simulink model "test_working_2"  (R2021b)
settings: Solver=FixedStepAuto  StartTime=0.0  StopTime=Inf  FixedStep=0.01  RelTol=1e-3  EnableMultiTasking=on
undefined symbols (not defined in the file): imu, localhost, name, type, value, vel
libraries: genomix x3

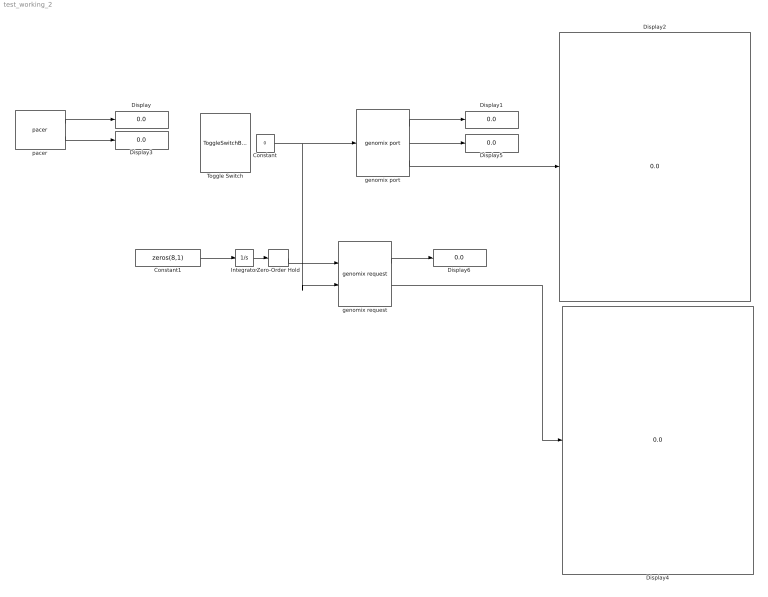
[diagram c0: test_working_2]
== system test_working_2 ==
  Constant : Constant  Value=0  OutDataTypeStr=boolean  SampleTime=-1
  Constant1 : Constant  Value=zeros(8,1)  OutDataTypeStr=double
  Display{,1..6} (7 alike) : Display
  Integrator : Integrator
  Toggle Switch : ToggleSwitchBlock
  Zero-Order Hold : ZeroOrderHold  SampleTime=-1
  genomix port : genomix/genomix port  host=localhost:20001  component=rotorcraft  instance=rotorcraft_mk3  port=imu  sigtype=value  timetype=triggered (level)  period=0.1  siglist="[{\"name\":\"imu.acc\",\"type\":\"value\",\"size\":3}]"
  genomix request : genomix/genomix request  host=localhost:20001  component=nhfc  instance=nhfc_mk3  port=set_state  sigtype=value  timetype=triggered (level)  period=Tsim  siglist="[{\"name\":\"vel\",\"type\":\"value\",\"size\":3}]"
  pacer : genomix/pacer  Priority=0  catchup=off
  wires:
  genomix port/1 -> Display1/1
  genomix port/3 -> Display2/1
  Constant/1 -> genomix request/2, genomix port/1
  pacer/1 -> Display/1
  pacer/2 -> Display3/1
  genomix request/2 -> Display4/1
  genomix port/2 -> Display5/1
  genomix request/1 -> Display6/1
  Constant1/1 -> Integrator/1
  Zero-Order Hold/1 -> genomix request/1
  Integrator/1 -> Zero-Order Hold/1
